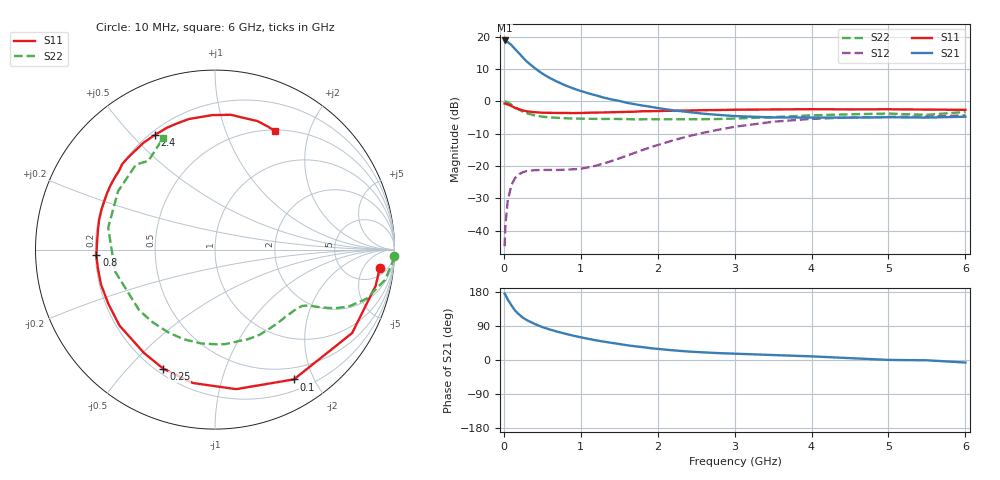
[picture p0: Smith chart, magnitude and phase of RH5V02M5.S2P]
! SIEMENS Small Signal Semiconductors
! BFR106
! Si NPN RF Bipolar Junction Transistor in SOT23
! VCE = 5 V  IC = 2.5 mA
! Common Emitter S-Parameters:  August  1996
# GHz  S  MA  R  50
!  f  S11  S21  S12  S22
! GHz  MAG  ANG  MAG  ANG  MAG  ANG  MAG  ANG
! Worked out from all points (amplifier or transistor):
!   36 points, 10 MHz to 6 GHz, reference 50 ohm
!   highest |S21| = 18.8 dB at 10 MHz (marker M1)
!   |S21| within 3 dB of that: start of sweep to 159 MHz
!   unconditionally stable (mu >= 1): 754.5 MHz to 1.836 GHz; 4.229 GHz to end of sweep
!   at 250 MHz: K = 0.35, MSG = 17.7 dB, |S12| = -21.9 dB
!   at 1.4 GHz: K = 1.22, MAG = 6.7 dB, |S12| = -18.4 dB
!   at 6 GHz: K = 1.02, MAG = -1.1 dB, |S12| = -4.3 dB
!   S11 on the Smith chart (normalised r, x): 10 MHz: 8, -12; 100 MHz: 0.34, -1.73; 250 MHz: 0.23, -0.63; 800 MHz: 0.20, -0.02; 2.4 GHz: 0.22, +0.58; 6 GHz: 0.52, +1.50
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0.01  0.9231 -6.5  8.708 175.3  0.0058 87.3  0.9975 -2.2
0.02  0.9178 -12.6  8.621 172.0  0.012 83.9  0.9914 -4.2
0.05  0.8944 -31.3  8.241 159.8  0.0289 73.0  0.9622 -10.1
0.1  0.8463 -58.7  7.37 143.8  0.0517 59.5  0.887 -18.0
0.15  0.7863 -81.4  6.324 129.5  0.0664 49.0  0.8076 -23.2
0.2  0.7534 -99.4  5.486 119.8  0.0751 42.5  0.7425 -26.1
0.25  0.7237 -113.4  4.713 111.3  0.0805 37.2  0.6892 -28.0
0.3  0.6988 -124.4  4.103 105.1  0.084 34.4  0.6551 -29.2
0.4  0.68 -141.5  3.271 95.2  0.0865 30.6  0.6061 -30.9
0.5  0.6665 -153.2  2.684 86.9  0.0871 29.9  0.5792 -32.8
0.6  0.6641 -162.9  2.285 80.3  0.0872 30.7  0.5647 -35.1
0.8  0.6617 -177.6  1.762 69.3  0.0879 36.0  0.5484 -40.7
1.1  0.6667 165.4  1.33 55.8  0.0956 49.9  0.537 -50.7
1.6  0.6872 144.7  0.949 39.0  0.1447 67.2  0.5315 -70.4
2.2  0.7161 124.0  0.726 25.5  0.2498 67.4  0.5288 -98.3
2.4  0.7216 117.6  0.683 22.3  0.2895 64.7  0.5291 -109.3
3.5  0.7495 91.2  0.564 13.1  0.4839 40.9  0.5701 -167.7
4  0.7564 83.3  0.561 9.6  0.536 29.3  0.6075 168.4
4.5  0.7509 77.1  0.56 4.9  0.5626 18.9  0.6305 148.9
5  0.7541 71.7  0.568 0.2  0.5762 10.3  0.6469 132.9
5.5  0.7457 66.4  0.561 -0.8  0.5808 6.1  0.6183 126.9
6  0.7391 63.1  0.579 -6.7  0.6068 -2.0  0.6867 114.7
